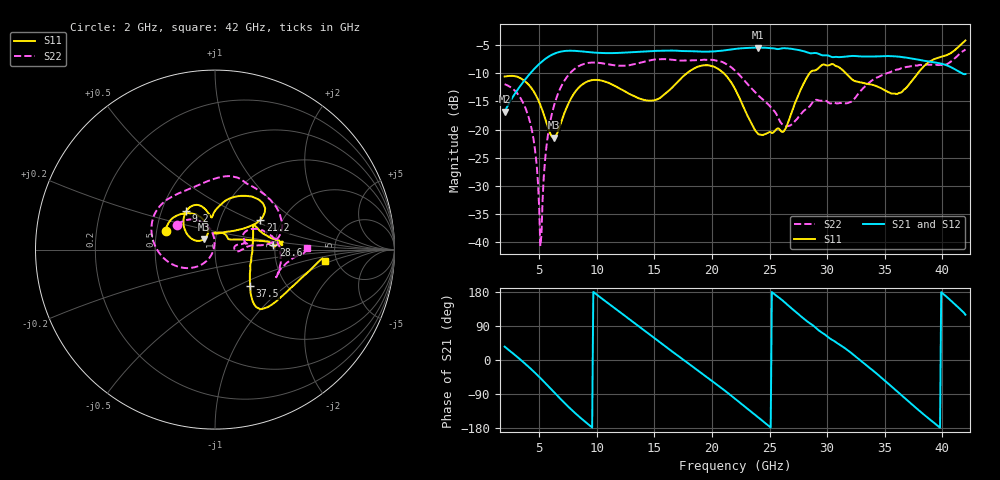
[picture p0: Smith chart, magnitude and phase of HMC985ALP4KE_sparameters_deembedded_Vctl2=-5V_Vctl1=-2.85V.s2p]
!s2p File: Measurements: S11, S21, S12, S22
# GHz S dB R 50.0
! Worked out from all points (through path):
!   401 points, 2 GHz to 42 GHz, reference 50 ohm
!   highest |S21| = -5.48 dB at 24 GHz (marker M1); lowest = -16.9 dB at 2 GHz (marker M2)
!   lowest |S11| = -21.5 dB at 6.3 GHz (marker M3), VSWR 1.18, Z = 44.1 + j5.31 ohm
!   |S11| at or under -10 dB: start of sweep to 17.84 GHz; 21.01 GHz to 28.49 GHz (7.476 GHz wide, 30.2 % of centre); 31.6 GHz to 37.89 GHz (6.284 GHz wide, 18.1 % of centre)
!   |S22| runs from -40.7 to -5.8 dB; largest |S21 - S12| = 0.00058
!   S11 on the Smith chart (normalised r, x): 2 GHz: 0.56, +0.13; 9.2 GHz: 0.67, +0.31; 21.2 GHz: 1.55, +0.57; 28.6 GHz: 1.95, +0.12; 37.5 GHz: 1.34, -0.59; 42 GHz: 4.02, -0.81
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2  -10.62 159.3  -16.87 35.3  -16.87 35.3  -11.96 146.8
4.1  -12.09 125.3  -10.35 -18.4  -10.35 -18.4  -17.92 105.3
4.6  -13.49 116.5  -9.21 -32.6  -9.21 -32.6  -22.95 95.4
5.1  -15.64 109.5  -8.21 -47.5  -8.21 -47.5  -40.67 132.8
5.7  -19.21 110.4  -7.25 -66.2  -7.25 -66.2  -21.89 -126.8
6.3  -21.45 135.0  -6.58 -85.3  -6.58 -85.3  -15.69 -141.9
8.7  -12.09 134.4  -6.17 -155.5  -6.17 -155.5  -8.52 160.8
9.2  -11.48 127.0  -6.27 -168.2  -6.27 -168.2  -8.23 152.3
12.7  -13.55 100.9  -6.35 110.7  -6.35 110.7  -8.65 105.8
15.4  -14.52 94.4  -6.06 48.7  -6.06 48.7  -7.55 76.3
18.1  -9.61 64.7  -6.11 -12.5  -6.11 -12.5  -7.76 56.9
21.2  -10.38 33.1  -5.95 -82.7  -5.95 -82.7  -8.37 15.3
22  -12.79 34.0  -5.73 -102.2  -5.73 -102.1  -9.56 7.9
24  -20.77 79.3  -5.49 -151.0  -5.49 -151.0  -13.91 6.4
26.3  -20.13 35.3  -5.59 152.5  -5.59 152.5  -19.31 1.8
28.6  -9.75 5.0  -6.50 94.9  -6.51 94.9  -15.59 12.3
28.7  -9.61 3.7  -6.49 92.9  -6.50 92.9  -15.28 12.3
32.4  -11.42 23.6  -6.98 10.9  -6.98 10.9  -14.48 30.1
35.4  -13.45 8.3  -6.99 -65.0  -6.99 -64.9  -9.90 14.3
37.5  -11.02 -45.9  -7.47 -120.9  -7.48 -120.9  -8.75 -3.8
39.8  -7.18 -46.0  -8.29 -178.6  -8.29 -178.5  -8.56 -23.4
42  -4.22 -5.9  -10.18 119.4  -10.19 119.4  -5.81 0.7
